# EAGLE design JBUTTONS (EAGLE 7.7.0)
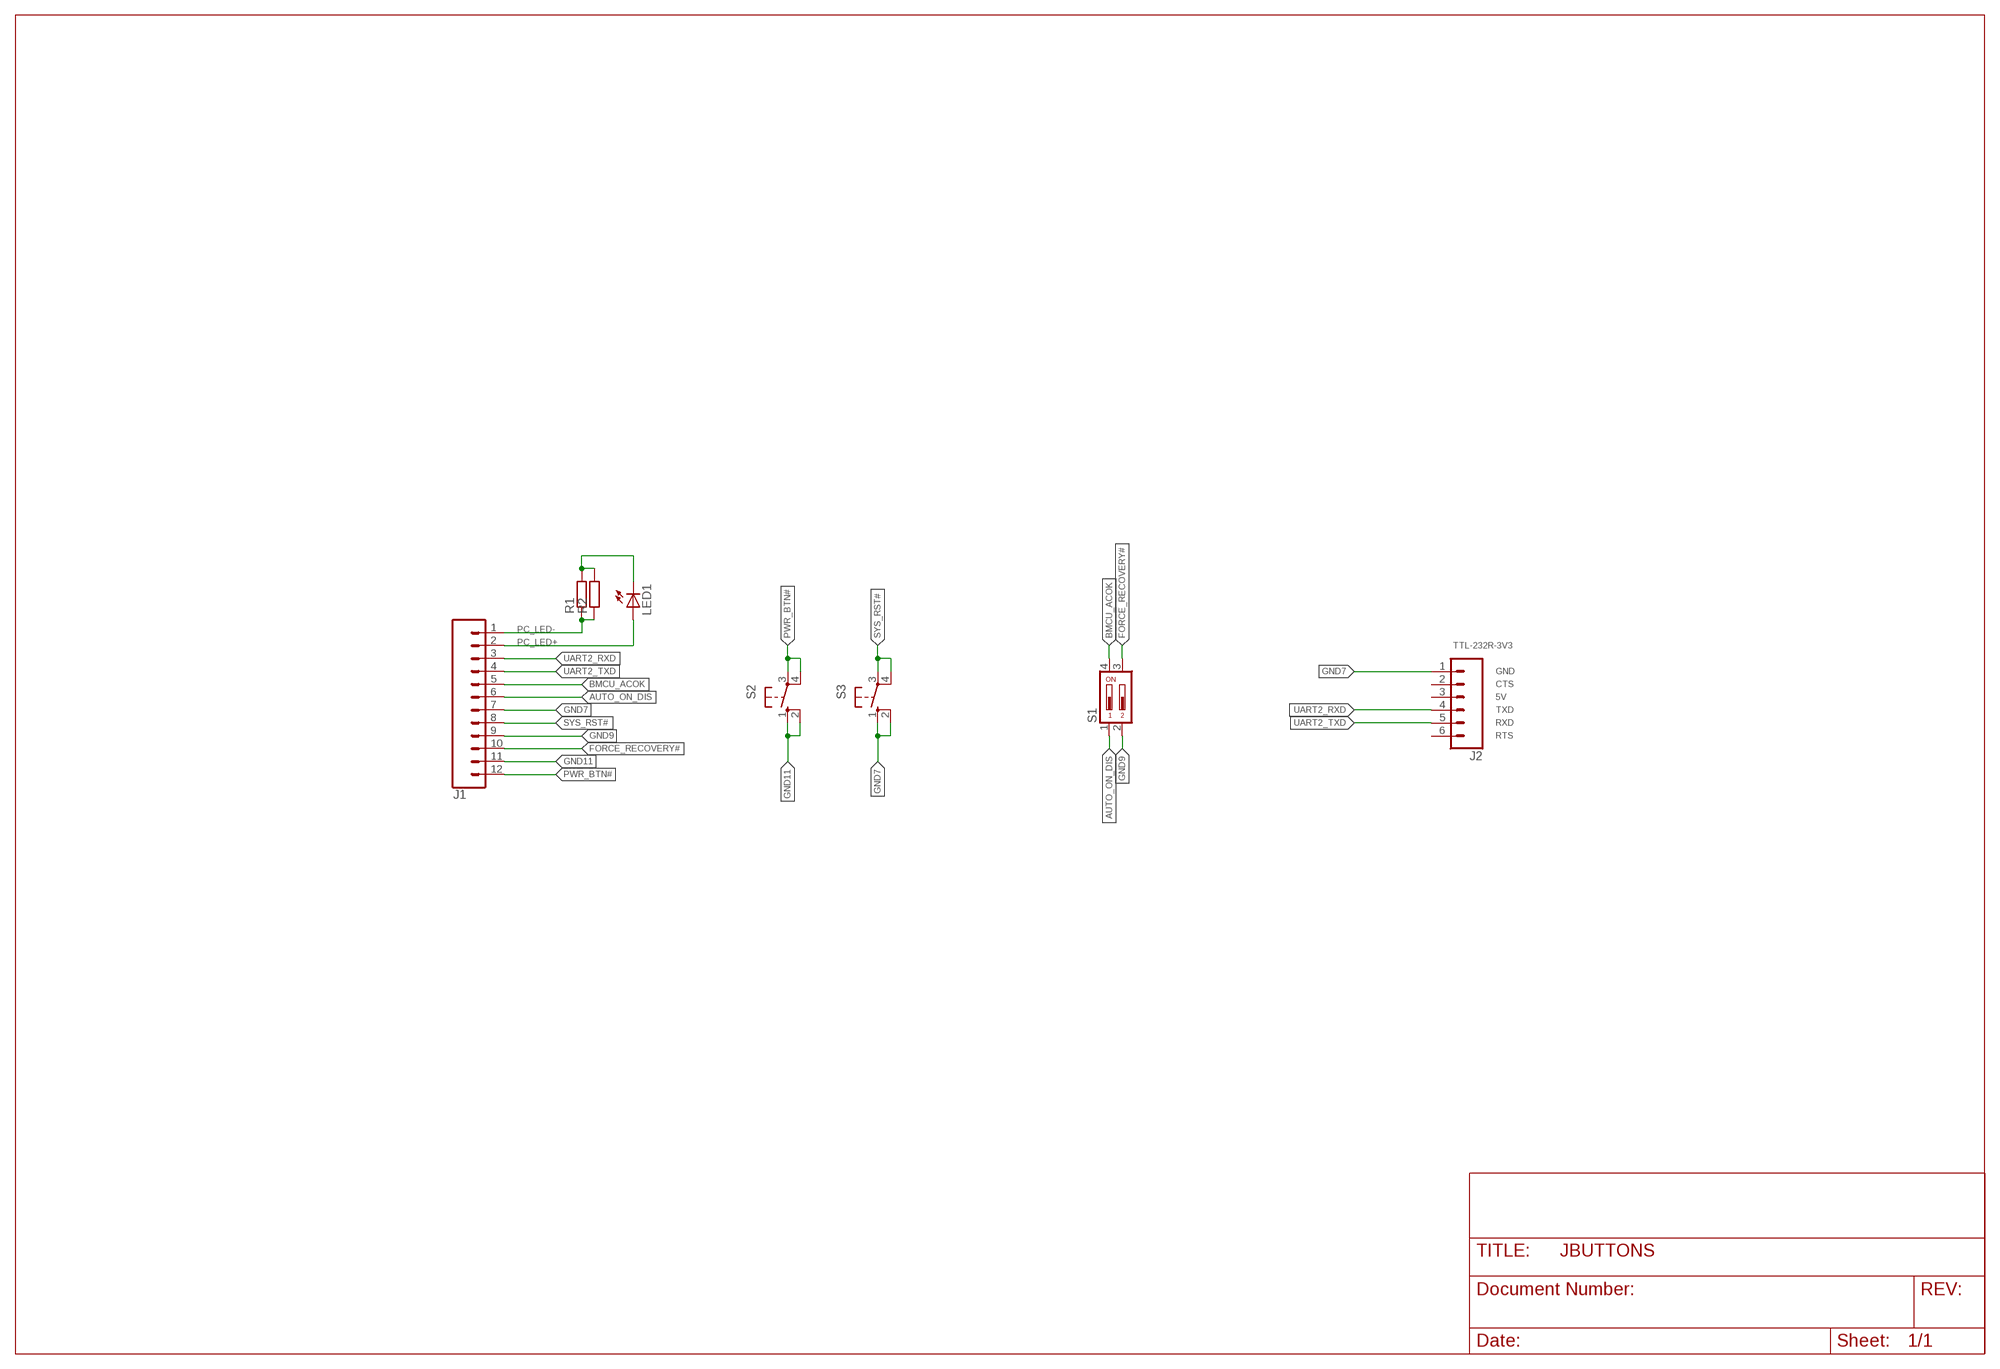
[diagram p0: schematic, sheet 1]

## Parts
J1  CONN_12LOCK_NO_SILK  [1X12_LOCK_NO_SILK]
J2  CONN_06LOCK  [1X06_LOCK]
LED1  LED5MM  [LED5MM]
R1  R-EU_0207/10  [0207/10]
R2  R-EU_R0603  [R0603]
S1  DS02  [DS-02]
S2  10-XX  [B3F-10XX]
S3  10-XX  [B3F-10XX]

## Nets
AUTO_ON_DIS: J1.6 S1.1
BMCU_ACOK: J1.5 S1.4
FORCE_RECOVERY#: J1.10 S1.3
GND7: J1.7 J2.1 S3.1(S) S3.2(S1)
GND9: J1.9 S1.2
GND11: J1.11 S2.1(S) S2.2(S1)
N$2: LED1.K(C) R1.2 R2.2
PC_LED+: J1.2 LED1.A
PC_LED-: J1.1 R1.1 R2.1
PWR_BTN#: J1.12 S2.3(P) S2.4(P1)
SYS_RST#: J1.8 S3.3(P) S3.4(P1)
UART2_RXD: J1.3 J2.4
UART2_TXD: J1.4 J2.5
Unconnected: J2.2 J2.3 J2.6

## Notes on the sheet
- TTL-232R-3V3
- GND
- CTS
- 5V
- TXD
- RXD
- RTS

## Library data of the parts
J1 = SparkFun-Connectors:CONN_12: Multi connection point. Often used as Generic Header-pin footprint for 0.1 inch spaced/style header connections On any of the 0.1 inch spaced packages, you can populate with these: Break Away Headers - Straight (PRT-00116) Break Away Male Headers - Right Angle (PRT-00553) Female Headers (PRT-00115)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
J2 = SparkFun-Connectors:CONN_06: Multi connection point. Often used as Generic Header-pin footprint for 0.1 inch spaced/style header connections On any of the 0.1 inch spaced packages, you can populate with these: Break Away Headers - Straight (PRT-00116) Break Away Male Headers - Right Angle (PRT-00553) Female Headers (PRT-00115)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
LED1 = led:LED: LED
R1 R2 = rcl:R-EU_: RESISTOR, European symbol
S1 = switch-dil:DS02: DIL/CODE SWITCH; OC_FARNELL: 9472126; OC_NEWARK: unknown
S2 S3 = switch-omron:10-XX: OMRON SWITCH; MPN: B3F-1000; OC_FARNELL: 176432; OC_NEWARK: 36M3542

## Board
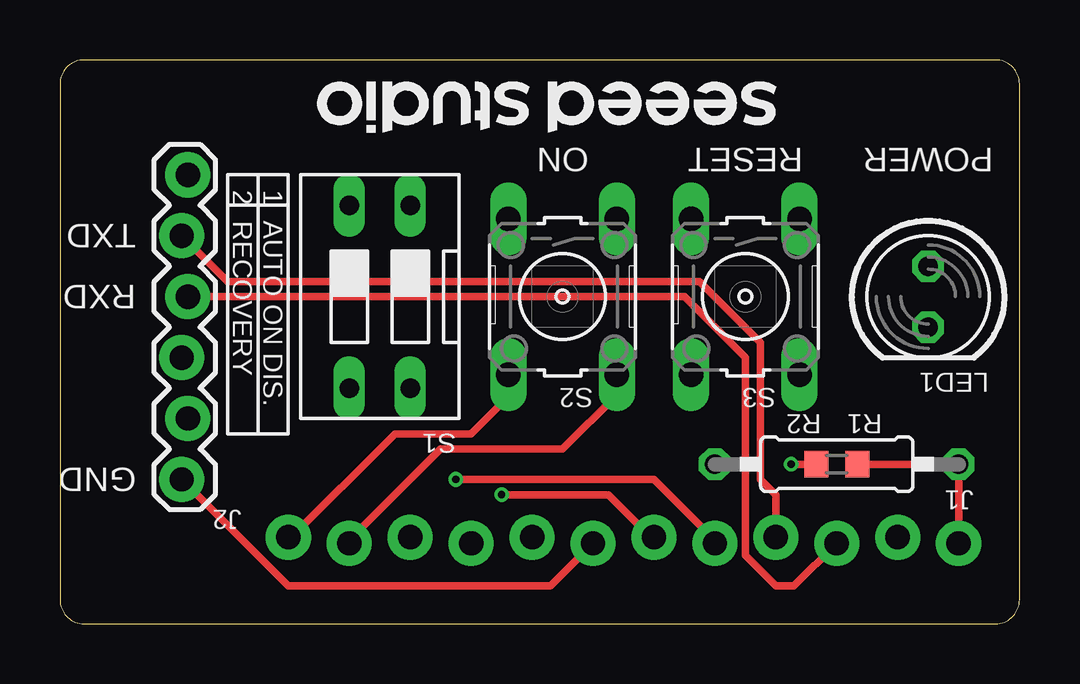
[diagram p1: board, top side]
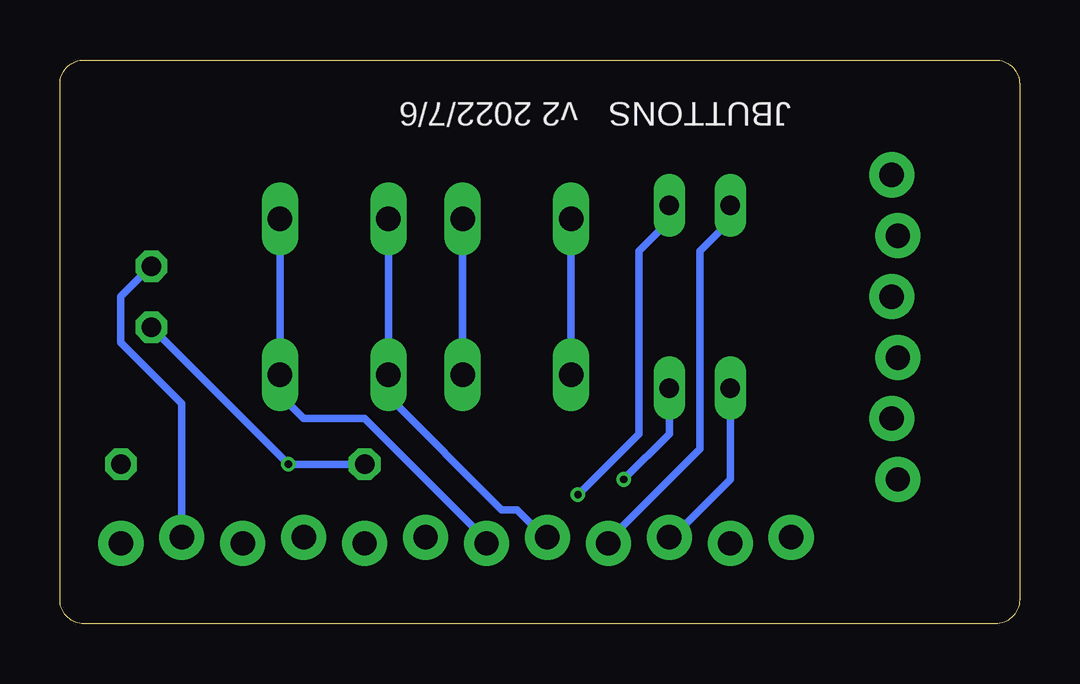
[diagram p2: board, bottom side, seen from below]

Size 40 x 23.51 mm. Coordinates in mm from the lower left corner, seen from the top.
Outline: 0,22.51 0,1 arc90 1,0 39,0 arc90 40,1 40,22.51 arc90 39,23.51 1,23.51 arc90 0,22.51
Copper layers (1*16): Top 0.035mm / dielectric 1.5mm / Bottom 0.035mm
Design rules "SeeedStudio_2layer_DRU_no_angle_20140221": minimum track width 6mil, minimum drill 12mil, track to track 6mil, track to pad 6mil, pad to pad 6mil, via to via 6mil, smd to smd 0mil, copper to edge 10mil, drill to drill 10mil, minimum pad ring 10mil, minimum via ring 6mil, stop-mask expansion 2mil, vias tented up to drill 100mil, thermal gap 10mil

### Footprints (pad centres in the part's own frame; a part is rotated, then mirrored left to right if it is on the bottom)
1X12_LOCK_NO_SILK = drill 1.016 pad 1.88: 1 0,0.127; 2 2.54,-0.127; 3 5.08,0.127; 4 7.62,-0.127; 5 10.16,0.127; 6 12.7,-0.127; 7 15.24,0.127; 8 17.78,-0.127; 9 20.32,0.127; 10 22.86,-0.127; 11 25.4,0.127; 12 27.94,-0.127
1X06_LOCK = drill 1.016 pad 1.88: 1 0,0; 2 2.54,-0.254; 3 5.08,0; 4 7.62,-0.254; 5 10.16,0; 6 12.7,-0.254
LED5MM = drill 0.813 octagon: A -1.27,0; K 1.27,0
0207/10 = drill 0.813 octagon: 1 -5.08,0; 2 5.08,0
R0603 = smd 1 x 1.1: 1 -0.85,0; 2 0.85,0
DS-02 = drill 0.813 long: 1 -1.27,-3.81; 2 1.27,-3.81; 3 1.27,3.81; 4 -1.27,3.81
B3F-10XX = drill 1.016 long: 1 -3.251,2.261; 2 3.251,2.261; 3 -3.251,-2.261; 4 3.251,-2.261

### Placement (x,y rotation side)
J1  37.46,3.48 180 top
J2  5.07,6.02 90 top
LED1  36.19,13.64 270 top
R1  32.38,6.65 180 top
R2  32.38,6.65 180 top
S1  13.33,13.64 180 top
S2  20.95,13.64 270 top
S3  28.57,13.64 270 top

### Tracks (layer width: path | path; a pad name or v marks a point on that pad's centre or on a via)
AUTO_ON_DIS  (via drill 0.3)
  Top 0.305: v18.41,5.38 22.86,5.38 24.76,3.48 J1.6
  Bottom 0.305: v18.41,5.38 15.87,7.93 15.87,15.54 14.6,16.82 S1.1
BMCU_ACOK  (via drill 0.3)
  Top 0.305: v16.5,6.02 24.76,6.02 27.3,3.48 J1.5
  Bottom 0.305: v16.5,6.02 14.6,7.93 S1.4
FORCE_RECOVERY#
  Bottom 0.305: S1.3 12.06,6.02 14.6,3.48 J1.10
GND7
  Top 0.305: J1.7 20.44,1.57 9.52,1.57 J2.1
  Bottom 0.305: S3.1 S3.2 30.83,9.55 29.84,8.56 27.3,8.56 22.22,3.48 J1.7
GND9
  Bottom 0.305: J1.9 17.14,3.48 13.33,7.29 13.33,15.54 12.06,16.82 S1.2
GND11
  Top 0.305: J1.11 12.06,3.48 15.87,7.29 20.95,7.29 23.21,9.55 S2.2
  Bottom 0.305: S2.2 S2.1
N$2  (via drill 0.3)
  Top 0.305: R2.2 v30.47,6.65
  Bottom 0.305: R1.2 v30.47,6.65 LED1.K
PC_LED+
  Bottom 0.305: J1.2 34.92,9.2 37.46,11.74 37.46,13.64 LED1.A
PC_LED-
  Top 0.305: J1.1 R1.1 R2.1
PWR_BTN#
  Top 0.305: J1.12 9.52,3.48 13.96,7.93 17.14,7.93 18.69,9.47 S2.4
  Bottom 0.305: S2.4 S2.3
SYS_RST#
  Bottom 0.305: J1.8 19.68,3.48 20.95,4.75 21.59,4.75 26.31,9.47 S3.4 S3.3
UART2_RXD
  Top 0.305: J1.3 30.6,1.57 29.84,1.57 28.57,2.84 28.57,11.1 26.03,13.64 J2.4
UART2_TXD
  Top 0.305: J1.4 29.84,5.38 29.2,6.02 29.2,11.74 26.66,14.28 6.98,14.28 J2.5

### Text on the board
tPlace: ON | RESET | POWER | 2 | 1 | TXD | RECOVERY | AUTO ON DIS. | RXD | GND
bPlace: JBUTTONS | v2 2022/7/6

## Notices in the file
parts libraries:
SparkFun-Connectors: Licensing: Creative Commons ShareAlike 4.0 International - https://creativecommons.org/licenses/by-sa/4.0
